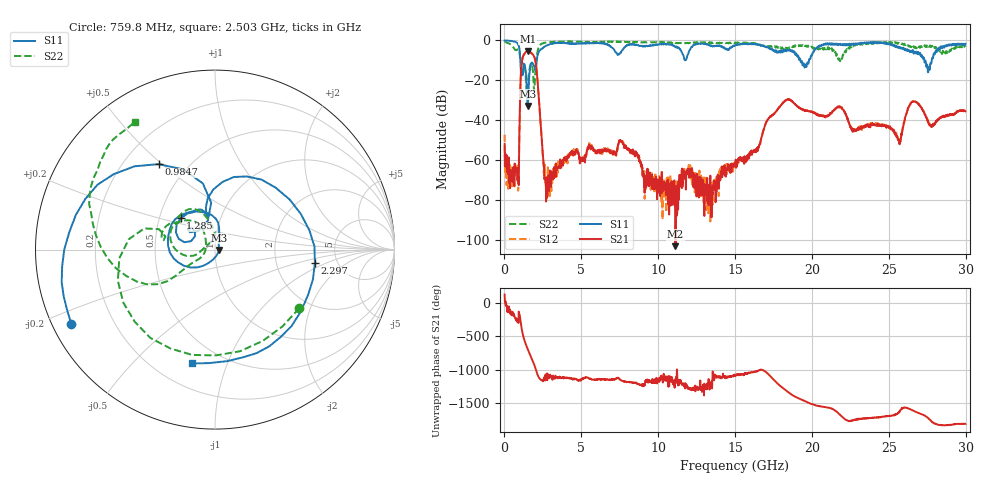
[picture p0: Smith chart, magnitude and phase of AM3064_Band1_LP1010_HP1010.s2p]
# Hz S DB R 50.0
!freq dBS11 angS11 dBS21 angS21 dBS12 angS12 dBS22 angS22
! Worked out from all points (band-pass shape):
!   1600 points, 10 MHz to 29.98 GHz, reference 50 ohm
!   highest |S21| = -5.31 dB at 1.51 GHz (marker M1); lowest = -103.1 dB at 11.13 GHz (marker M2)
!   |S21| within 3 dB of the highest: 1.196 GHz to 1.941 GHz (745.6 MHz wide, 47.5 % of centre)
!   lowest |S11| = -32.9 dB at 1.51 GHz (marker M3), VSWR 1.05, Z = 52.3 - j0.184 ohm
!   |S11| at or under -10 dB: 1.031 GHz to 2.103 GHz (1.071 GHz wide, 68.4 % of centre); 19.25 GHz to 19.81 GHz (555.5 MHz wide, 2.84 % of centre); 27.3 GHz to 27.79 GHz (488 MHz wide, 1.77 % of centre)
!   |S22| runs from -26.6 to -0.4 dB; largest |S21 - S12| = 0.0059
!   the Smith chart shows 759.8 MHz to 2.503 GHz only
!   S11 on the Smith chart (normalised r, x): 759.8 MHz: 0.06, -0.24; 984.7 MHz: 0.35, +0.49; 1.285 GHz: 0.64, +0.24; 2.297 GHz: 3.38, -0.75; 2.503 GHz: 0.35, -0.76
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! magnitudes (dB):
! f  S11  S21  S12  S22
! 10 MHz  0.0  -51.9  -47.2  -0.4
! 759.8 MHz  -0.9  -65.3  -64.3  -4.9
! 984.7 MHz  -4.9  -40.9  -40.8  -6.3
! 1.135 GHz  -14.9  -10.7  -10.6  -10.8
! 1.285 GHz  -11.7  -6.9  -6.8  -11.4
! 1.51 GHz  -32.9  -5.3  -5.3  -22.7
! 1.978 GHz  -14.1  -9.1  -9.1  -19.8
! 2.297 GHz  -5.0  -35.6  -35.6  -2.4
! 2.503 GHz  -3.8  -57.6  -58.5  -1.5
! 2.784 GHz  -2.4  -78.5  -71.3  -1.0
! 5.015 GHz  -1.4  -59.1  -59.0  -0.8
! 7.582 GHz  -6.1  -50.3  -50.7  -0.7
! 10 GHz  -2.0  -70.0  -74.2  -1.0
! 11.13 GHz  -3.4  -103.1  -78.9  -1.2
! 15 GHz  -2.6  -61.9  -63.0  -1.4
! 18.29 GHz  -4.6  -30.2  -30.2  -4.0
! 19.99 GHz  -7.6  -35.8  -35.9  -3.2
! 25 GHz  -1.4  -43.7  -43.3  -1.1
! 25.69 GHz  -3.5  -51.7  -50.5  -1.6
! 26.63 GHz  -6.6  -30.5  -30.5  -3.1
! 27.56 GHz  -16.0  -40.4  -40.5  -2.6
! 29.98 GHz  -1.7  -35.5  -35.1  -3.1
